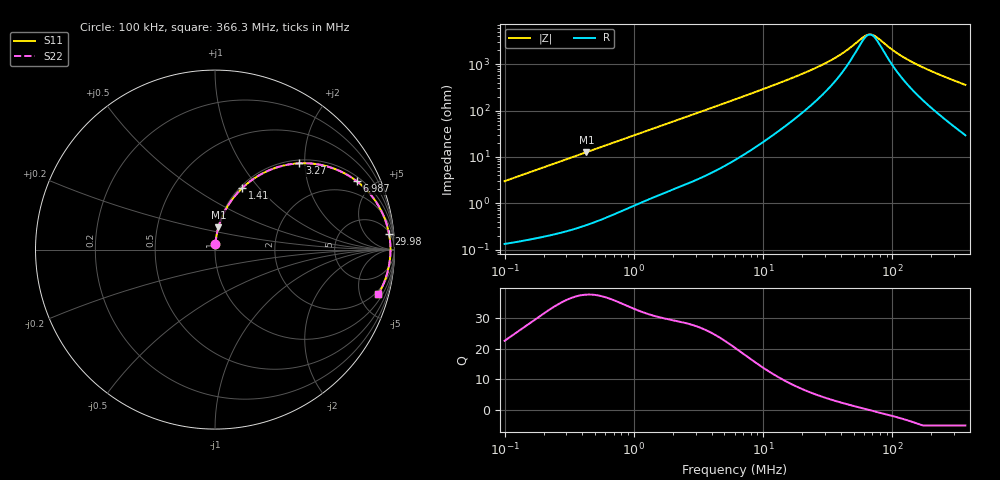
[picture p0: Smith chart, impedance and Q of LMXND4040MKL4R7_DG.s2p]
! LMXND4040MKL4R7_DG  S-PARAMETER MODEL  ( General Type )
! Model Generated by TAIYO YUDEN Corporation (https://www.yuden.co.jp/en/)
! Version 1.0
! TAIYO YUDEN Control No. 191023NI43SB-FBB
! Copyright(c) 2019 TAIYO YUDEN CO.,LTD. All Rights Reserved.
! Product Description (link to TY-COMPAS)
! https://ds.yuden.co.jp/TYCOMPAS/or/detail?pn=LMXND4040MKL4R7MDG&u=M
! Products Name : Inductors
! Characteristics :
!  Inductance : 4.7 uH , SRF(min) : 45 MHz , DC Resistance(max) : 0.114 Ohm
!  Rated Current : Saturation :1200 mA , Temp Rise : 1500 mA (40 degC)
!  Case Size : 4.0 x 4.0 / 0.157 x 0.157 [mm/inch] , Thickness : 1.2 / 0.047 [mm/inch]
!  (Conditions: Temperature = 25 degC , DC Bias Current/Voltage = 0A / 0V)
! External Node Assignments :
!  1  o---GGG---o  2
! GND o---------o GND
! Frequency Range : 0.1MHz  -  366.261039MHz  [ 402 STEP ]
# MHz S RI R 50
! Freq[MHz].  S11 Real  S11 Imag  S21 Real  S21 Imag  S12 Real  S12 Imag  S22 Real  S22 Imag
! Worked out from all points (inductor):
!   401 points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, 100 kHz to 366.3 MHz, reference 50 ohm
!   read as one part in series: L = 4.76 uH near 104.2 kHz
!   highest Q = 37.7 at 429.1 kHz (marker M1), where L = 4.7 uH
!   self-resonance near 66.87 MHz
!   S11 on the Smith chart (normalised r, x): 100 kHz: 1.00, +0.06; 1.41 MHz: 1.03, +0.82; 3.27 MHz: 1.07, +1.88; 6.987 MHz: 1.22, +4.02; 29.98 MHz: 6, +20; 366.3 MHz: 1.59, -7.14
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0.1  0.00222 0.0299  0.9978 -0.0299  0.9978 -0.0299  0.00222 0.0299
0.395307  0.0164 0.1146  0.9836 -0.1146  0.9836 -0.1146  0.0164 0.1146
0.429114  0.019 0.1239  0.981 -0.1239  0.981 -0.1239  0.019 0.1239
0.844473  0.0636 0.23  0.9364 -0.23  0.9364 -0.23  0.0636 0.23
1.410336  0.1517 0.3428  0.8483 -0.3428  0.8483 -0.3428  0.1517 0.3428
1.562679  0.1783 0.3666  0.8217 -0.3666  0.8217 -0.3666  0.1783 0.3666
3.270477  0.4697 0.4808  0.5303 -0.4808  0.5303 -0.4808  0.4697 0.4808
4.448906  0.615 0.4663  0.385 -0.4663  0.385 -0.4663  0.615 0.4663
6.177387  0.7487 0.4096  0.2513 -0.4096  0.2513 -0.4096  0.7487 0.4096
6.986533  0.7894 0.3815  0.2106 -0.3815  0.2106 -0.3815  0.7894 0.3815
11.9099  0.9061 0.2524  0.0939 -0.2524  0.0939 -0.2524  0.9061 0.2524
23.92381  0.9624 0.1204  0.0376 -0.1204  0.0376 -0.1204  0.9624 0.1204
29.9802  0.9694 0.0887  0.0306 -0.0887  0.0306 -0.0887  0.9694 0.0887
40.78277  0.9749 0.0515  0.0251 -0.0515  0.0251 -0.0515  0.9749 0.0515
58.99936  0.9776 0.0126  0.0224 -0.0126  0.0224 -0.0126  0.9776 0.0126
64.045  0.9777 0.00432  0.0223 -0.00432  0.0223 -0.00432  0.9777 0.00432
68.11043  0.9777 -0.00186  0.0223 0.00186  0.0223 0.00186  0.9777 -0.00186
73.93525  0.9776 -0.0101  0.0224 0.0101  0.0224 0.0101  0.9776 -0.0101
94.57258  0.9765 -0.0355  0.0235 0.0355  0.0235 0.0355  0.9765 -0.0355
120.9704  0.9737 -0.0628  0.0263 0.0628  0.0263 0.0628  0.9737 -0.0628
161.2173  0.9676 -0.0992  0.0324 0.0992  0.0324 0.0992  0.9676 -0.0992
366.261  0.9104 -0.2475  0.0896 0.2475  0.0896 0.2475  0.9104 -0.2475
